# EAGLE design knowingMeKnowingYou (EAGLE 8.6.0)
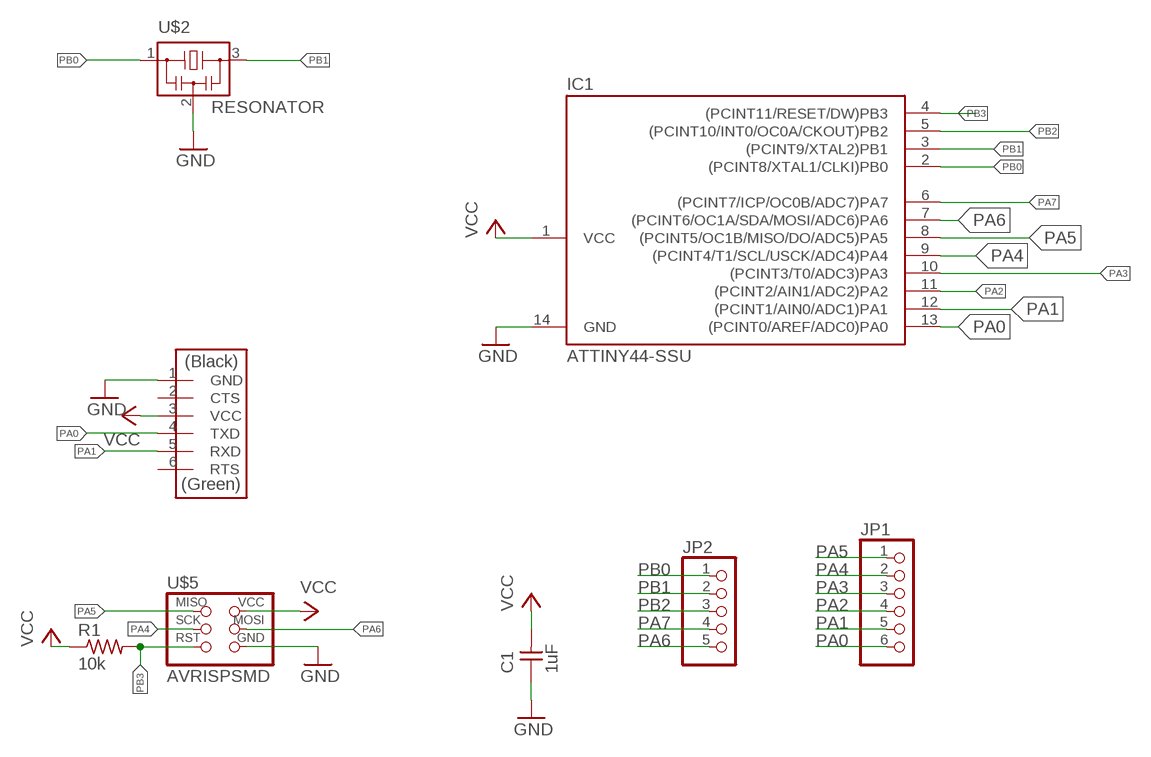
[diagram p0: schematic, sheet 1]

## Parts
C1  1uF  CAP-UNPOLARIZEDFAB  [C1206FAB]
IC1  ATTINY44-SSU  [SOIC14]
JP1  PINHD-1X06_2.54-SMD  [1X06SMD]
JP2  PINHD-1X05_2.54-SMD  [1X05SMD]
R1  10k  RES-US1206FAB  [R1206FAB]
U$2  RESONATOR  [EFOBM]
U$3  FTDI-SMD-HEADER  [1X06SMD]
U$5  AVRISPSMD  [2X03SMD]

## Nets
GND: C1.1 IC1.14(GND) U$2.2 U$3.1(GND) U$5.6(GND)
PA0: IC1.13((PCINT0/AREF/ADC0)PA0) JP1.6 U$3.4(TXD)
PA1: IC1.12((PCINT1/AIN0/ADC1)PA1) JP1.5 U$3.5(RXD)
PA2: IC1.11((PCINT2/AIN1/ADC2)PA2) JP1.4
PA3: IC1.10((PCINT3/T0/ADC3)PA3) JP1.3
PA4: IC1.9((PCINT4/T1/SCL/USCK/ADC4)PA4) JP1.2 U$5.3(SCK)
PA5: IC1.8((PCINT5/OC1B/MISO/DO/ADC5)PA5) JP1.1 U$5.1(MISO)
PA6: IC1.7((PCINT6/OC1A/SDA/MOSI/ADC6)PA6) JP2.5 U$5.4(MOSI)
PA7: IC1.6((PCINT7/ICP/OC0B/ADC7)PA7) JP2.4
PB0: IC1.2((PCINT8/XTAL1/CLKI)PB0) JP2.1 U$2.1
PB1: IC1.3((PCINT9/XTAL2)PB1) JP2.2 U$2.3
PB2: IC1.5((PCINT10/INT0/OC0A/CKOUT)PB2) JP2.3
PB3: IC1.4((PCINT11/RESET/DW)PB3) R1.2 U$5.5(RST)
VCC: C1.2 IC1.1(VCC) R1.1 U$3.3(VCC) U$5.2(VCC)
Unconnected: U$3.2(CTS) U$3.6(RTS)

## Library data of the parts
C1 = fab:CAP-UNPOLARIZED
IC1 = fab:ATTINY44
JP1 = pinhead-2:PINHD-1X06: PIN HEADER
JP2 = pinhead-2:PINHD-1X05: PIN HEADER
R1 = fab:RES-US: Resistor (US Symbol)
U$2 = fab:RESONATOR
U$3 = fab:FTDI-SMD-HEADER
U$5 = fab:AVRISP

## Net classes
0 default: width 0.3 mm, clearance 0.4 mm

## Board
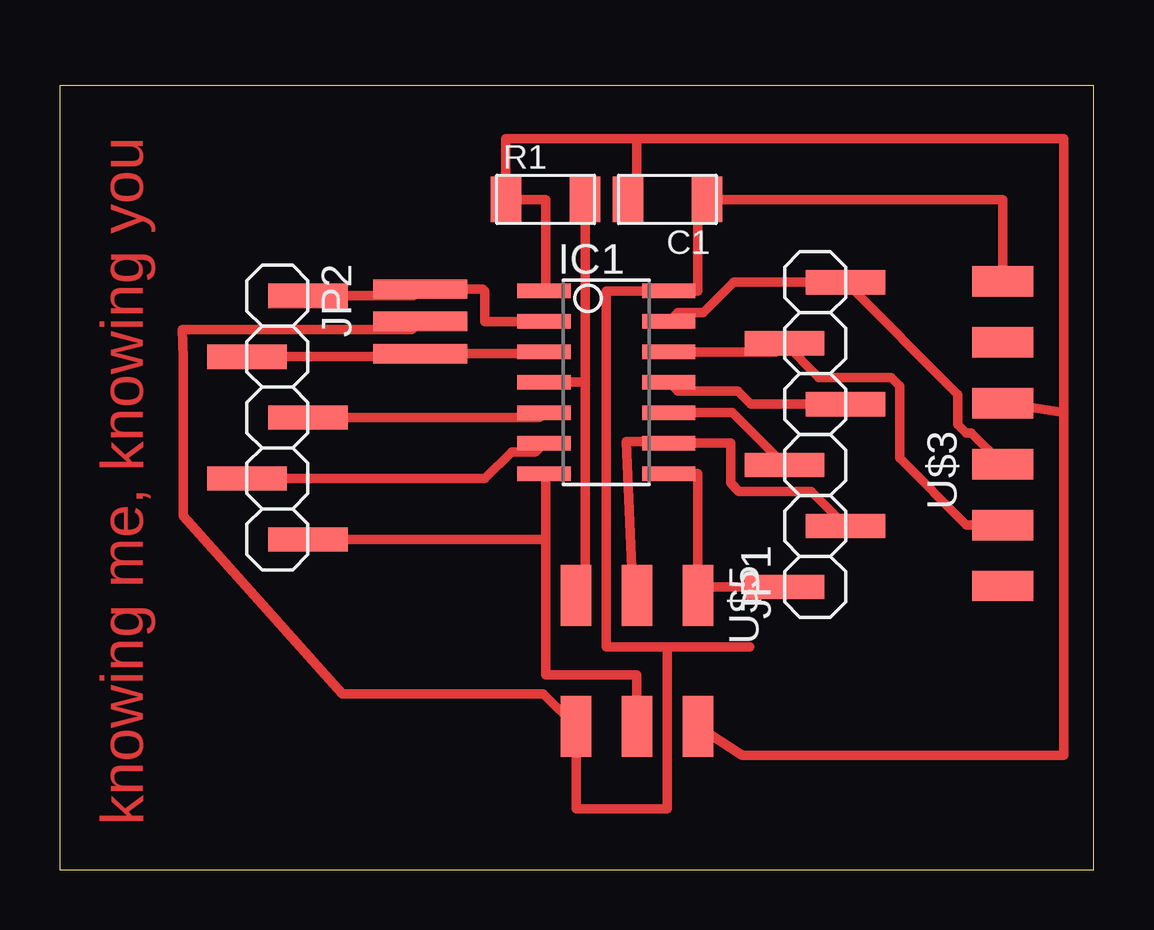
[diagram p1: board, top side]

Size 43.07 x 32.69 mm. Coordinates in mm from the lower left corner, seen from the top.
Outline: 0,0 43.07,0 43.07,32.69 0,32.69 0,0
Copper layers (1*16): Top 0.035mm / dielectric 1.5mm / Bottom 0.035mm
Design rules "default *": minimum track width 0.3mm, minimum drill 0.8mm, track to track 0.4mm, track to pad 0.4mm, pad to pad 0.4mm, via to via 0.4mm, smd to smd 6mil, copper to edge 40mil, drill to drill 6mil, minimum pad ring 10mil, minimum via ring 8mil, stop-mask expansion 4mil, vias tented up to drill 0mil, thermal gap 10mil

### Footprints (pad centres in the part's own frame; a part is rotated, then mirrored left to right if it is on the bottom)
C1206FAB = smd 1.27 x 1.905: 1 -1.651,0; 2 1.651,0
SOIC14 = smd 0.61 x 2.21: 1 -3.81,-2.603; 2 -2.54,-2.603; 3 -1.27,-2.603; 4 0,-2.603; 5 1.27,-2.603; 6 2.54,-2.603; 7 3.81,-2.603; 8 3.81,2.603; 9 2.54,2.603; 10 1.27,2.603; 11 0,2.603; 12 -1.27,2.603; 13 -2.54,2.603; 14 -3.81,2.603
1X06SMD = smd 1.016 x 3.302: 1 -1.27,1.27; 2 1.27,-1.27; 3 3.81,1.27; 4 6.35,-1.27; 5 8.89,1.27; 6 11.43,-1.27
1X05SMD = smd 1.016 x 3.302: 1 -1.27,1.27; 2 1.27,-1.27; 3 3.81,1.27; 4 6.35,-1.27; 5 8.89,1.27
R1206FAB = smd 1.27 x 1.905: 1 -1.651,0; 2 1.651,0
EFOBM = smd 0.8 x 3.9: 1 -1.35,0; 2 0,0; 3 1.35,0
1X06SMD' = smd 2.54 x 1.27: 1 0,6.35; 2 0,3.81; 3 0,1.27; 4 0,-1.27; 5 0,-3.81; 6 0,-6.35
2X03SMD = smd 2.54 x 1.27: 1 -2.54,2.54; 2 2.92,2.54; 3 -2.54,0; 4 2.92,0; 5 -2.54,-2.54; 6 2.92,-2.54

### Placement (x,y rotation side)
C1  25.31,27.94 180 top
IC1  22.77,20.32 270 top
JP1  31.46,13.06 90 top
JP2  9.06,22.66 270 top
R1  20.23,27.94 0 top
U$2  15.01,22.86 270 top
U$3  FTDI-SMD-HEADER  [1X06SMD']  39.28,18.18 0 top
U$5  24.04,8.89 270 top

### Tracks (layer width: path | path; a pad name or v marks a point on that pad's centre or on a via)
GND
  Top 0.4: U$3.1 39.28,27.94 C1.1 26.58,27.56 26.58,24.13 IC1.14 22.77,24.13 22.77,9.29 25.31,9.29 | 25.31,2.54 25.31,2.66 | 25.31,2.66 25.31,9.29 | 28.74,9.29 25.31,9.29 | 25.31,2.66 25.19,2.54 21.5,2.54 U$5.6 20.14,7.33 11.76,7.33 5.14,14.75 5.14,21.35 5.1,22.51 14.66,22.51 U$2.2
PA0
  Top 0.4: IC1.13 25.74,23.22 26.81,23.22 28.07,24.49 JP1.6 37.41,19.81 37.41,18.57 37.76,18.21 37.98,18.21 U$3.4
PA1
  Top 0.4: IC1.12 29.83,21.59 JP1.5 31.62,20.52 34.63,20.52 34.98,20.17 34.98,17.16 37.77,14.37 U$3.5
PA2
  Top 0.4: IC1.11 25.74,19.95 28.24,19.95 28.78,19.41 JP1.4
PA3
  Top 0.4: JP1.3 28.01,19.05 IC1.10
PA4
  Top 0.4: U$5.3 23.86,11.61 23.59,17.86 25.29,17.86 IC1.9 27.94,17.78 27.94,16.11 28.29,15.76 31.3,15.76 JP1.2
PA5
  Top 0.4: IC1.8 26.58,16.51 U$5.1 26.94,11.79 JP1.1
PA6
  Top 0.4: 20.23,13.86 20.23,16.45 IC1.7 | 20.23,13.86 20.23,8.13 24.04,8.13 U$5.4 | JP2.5 20.14,13.77 20.23,13.86
PA7
  Top 0.4: IC1.6 19.8,17.41 18.81,17.41 17.71,16.31 JP2.4
PB0
  Top 0.4: IC1.2 17.69,22.86 17.69,24.13 17.61,24.21 U$2.1 14.73,23.93 JP2.1
PB1
  Top 0.4: JP2.2 14.89,21.39 U$2.3 20.09,21.51 IC1.3
PB2
  Top 0.4: JP2.3 19.97,18.85 IC1.5
PB3
  Top 0.4: R1.2 21.88,20.32 | 21.88,20.32 21.88,12.26 | 21.88,12.26 21.88,11.81 | IC1.4 21.88,20.32 | U$5.5 21.5,11.88 21.88,12.26
VCC
  Top 0.4: 24.04,30.48 24.04,28.32 C1.2 | 24.04,30.48 18.58,30.48 R1.1 20.23,27.94 20.23,24.19 IC1.1 | 41.82,19.05 41.82,4.77 28.43,4.77 U$5.2 | 41.82,19.05 41.82,30.48 24.04,30.48 | U$3.3 41.82,19.05

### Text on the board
Top: knowing me, knowing you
